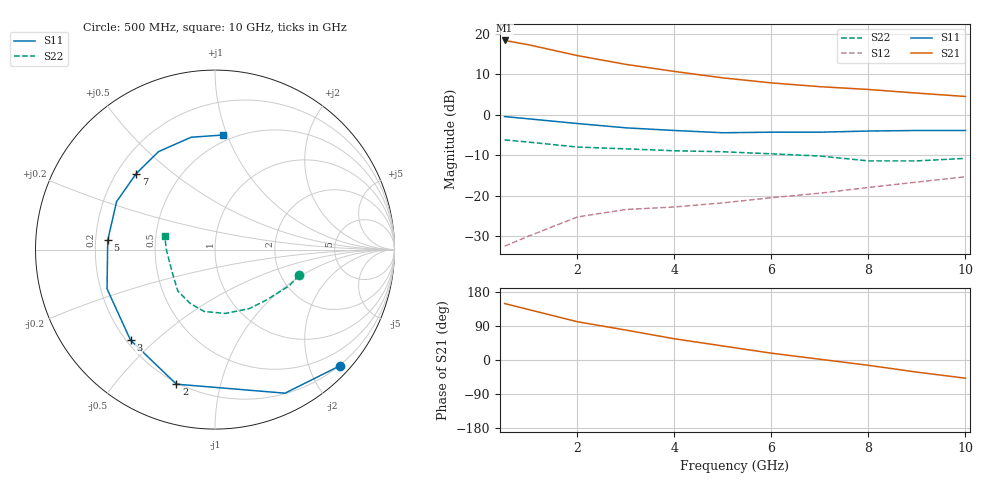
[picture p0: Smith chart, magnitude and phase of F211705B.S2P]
!ATF-21170
!S-PARAMETERS at Vds=5V  Id=80mA.  LAST UPDATED 07-22-92
# ghz s ma r 50
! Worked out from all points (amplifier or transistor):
!   11 points, 500 MHz to 10 GHz, reference 50 ohm
!   highest |S21| = 18.3 dB at 500 MHz (marker M1)
!   |S21| within 3 dB of that: start of sweep to 1.724 GHz
!   unconditionally stable (mu >= 1): 4.277 GHz to 9.245 GHz
!   at 1 GHz: K = 0.38, MSG = 23.6 dB, |S12| = -29.9 dB
!   at 5 GHz: K = 1.11, MAG = 13.4 dB, |S12| = -21.7 dB
!   at 10 GHz: K = 0.96, MSG = 9.9 dB, |S12| = -15.3 dB
!   S11 on the Smith chart (normalised r, x): 500 MHz: 0.19, -2.53; 2 GHz: 0.19, -0.74; 3 GHz: 0.22, -0.42; 5 GHz: 0.25, +0.04; 7 GHz: 0.28, +0.38; 10 GHz: 0.45, +0.97
0.5  0.95 -43.0  8.24 149.0  0.024 67.0  0.49 -17.0
1  0.89 -64.0  7.28 133.0  0.032 59.0  0.46 -26.0
2  0.78 -106.0  5.36 101.0  0.055 44.0  0.4 -45.0
3  0.69 -133.0  4.18 79.0  0.068 34.0  0.38 -60.0
4  0.64 -160.0  3.42 56.0  0.073 31.0  0.36 -81.0
5  0.6 175.0  2.85 37.0  0.082 24.0  0.35 -100.0
6  0.61 154.0  2.47 18.0  0.095 19.0  0.33 -115.0
7  0.61 136.0  2.22 2.0  0.108 12.0  0.31 -132.0
8  0.63 120.0  2.05 -14.0  0.127 7.0  0.27 -152.0
9  0.64 102.0  1.85 -32.0  0.148 0.0  0.27 -179.0
10  0.64 86.0  1.68 -48.0  0.172 -13.0  0.29 165.0
